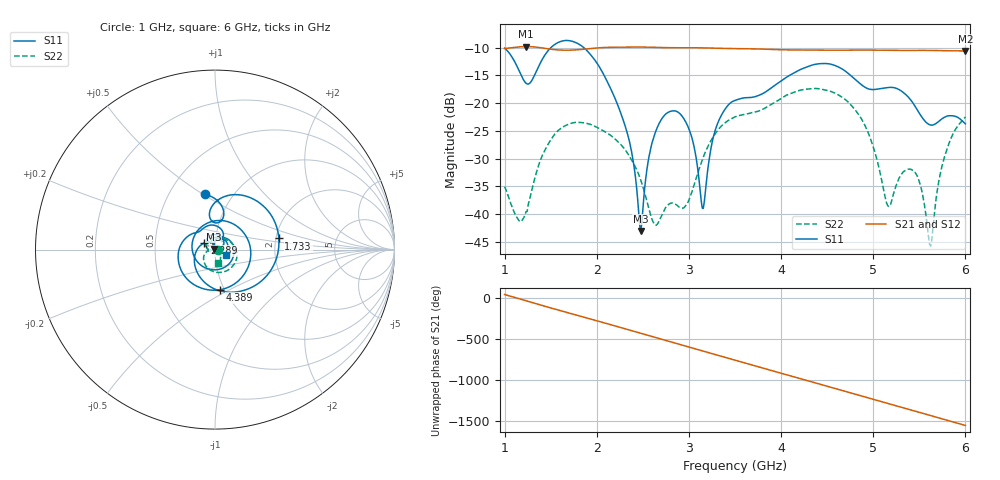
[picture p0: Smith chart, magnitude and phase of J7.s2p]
!Agilent Technologies,E8364B,MY43040528,A.07.50.67
!Agilent E8364B: A.07.50.67
!Date: Sunday, March 01, 2026 19:07:05
!Correction: S11(Full 2 Port(1,2))
!S21(Full 2 Port(1,2))
!S12(Full 2 Port(1,2))
!S22(Full 2 Port(1,2))
!S2P File: Measurements: S11, S21, S12, S22:
# Hz S  dB  R 50
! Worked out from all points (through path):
!   451 points, 1 GHz to 6 GHz, reference 50 ohm
!   highest |S21| = -9.79 dB at 1.233 GHz (marker M1); lowest = -10.6 dB at 6 GHz (marker M2)
!   group delay of S21, straight-line fit = 889 ps
!   lowest |S11| = -43.0 dB at 2.478 GHz (marker M3), VSWR 1.01, Z = 49.4 + j0.391 ohm
!   |S11| at or under -10 dB: start of sweep to 1.501 GHz; 1.86 GHz to end of sweep
!   |S22| runs from -45.8 to -17.3 dB; largest |S21 - S12| = 0.0014
!   S11 on the Smith chart (normalised r, x): 1 GHz: 0.74, +0.51; 1.733 GHz: 2.08, +0.30; 2.289 GHz: 0.89, +0.07; 4.389 GHz: 0.95, -0.45; 6 GHz: 1.12, -0.06
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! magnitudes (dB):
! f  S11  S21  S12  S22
! 1 GHz  -10.1  -10.1  -10.2  -35.0
! 1.156 GHz  -14.1  -9.9  -9.9  -41.1
! 1.233 GHz  -16.4  -9.8  -9.8  -39.5
! 1.444 GHz  -11.1  -10.1  -10.2  -28.2
! 1.733 GHz  -8.8  -10.4  -10.5  -23.6
! 1.844 GHz  -9.8  -10.3  -10.3  -23.5
! 2.289 GHz  -23.1  -9.9  -9.9  -28.0
! 2.478 GHz  -43.0  -9.9  -9.9  -33.9
! 2.567 GHz  -29.6  -9.9  -9.9  -39.1
! 2.667 GHz  -24.0  -10.0  -10.0  -41.5
! 2.956 GHz  -23.1  -10.0  -10.0  -38.7
! 3.156 GHz  -39.0  -10.0  -10.1  -29.8
! 3.289 GHz  -24.7  -10.1  -10.1  -25.4
! 3.5 GHz  -19.5  -10.2  -10.2  -22.5
! 4.344 GHz  -13.1  -10.4  -10.5  -17.4
! 4.389 GHz  -12.9  -10.4  -10.5  -17.4
! 4.867 GHz  -16.6  -10.4  -10.5  -22.7
! 5.167 GHz  -17.2  -10.5  -10.5  -38.6
! 5.433 GHz  -20.0  -10.5  -10.5  -32.1
! 5.622 GHz  -23.9  -10.5  -10.5  -45.8
! 5.767 GHz  -22.6  -10.5  -10.6  -30.1
! 6 GHz  -23.7  -10.6  -10.6  -22.5
